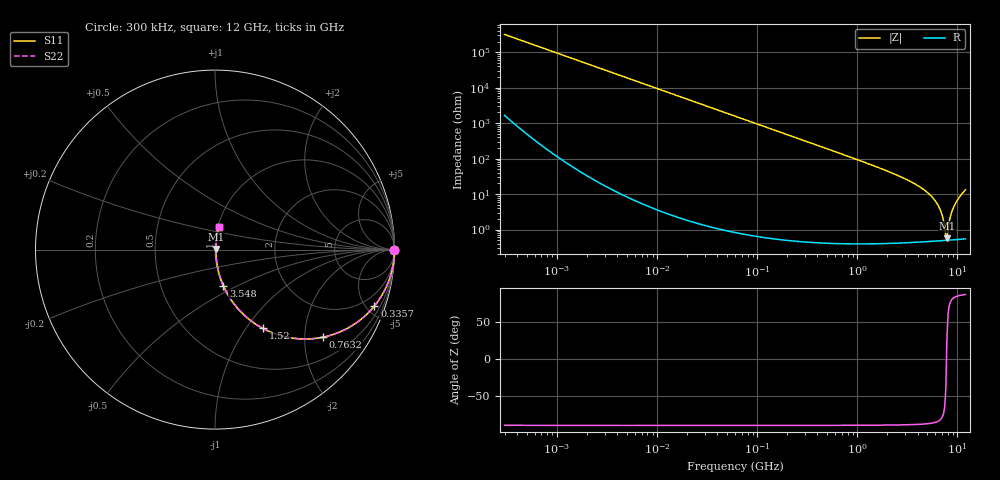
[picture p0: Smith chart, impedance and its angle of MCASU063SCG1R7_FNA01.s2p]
! MCASU063SCG1R7_FNA01  S-PARAMETER MODEL  ( General Type )
! Model Generated by TAIYO YUDEN Corporation (http://www.ty-top.com)
! Version 1.0
! TAIYO YUDEN Control No. 130801
! Copyright(c) 2013 TAIYO YUDEN CO.,LTD. All Rights Reserved.
! Product Description (link to TY-COMPAS)
! https://ds.yuden.co.jp/TYCOMPAS/or/detail?pn=MCASU063SCG1R7CFNA01&u=M
! Products Name : Multilayer Ceramic Capacitors
! Characteristics :
!  Capacitance : 1.7 pF , Rated Voltage : 50V , TCC : CG / C0G
!  Case Size : 0.6 x 0.3 / 0.024 x 0.012 [mm/inch] , Thickness : 0.3 / 0.012 [mm/inch]
!  (Conditions: Temperature = 25 degC , DC Bias Current/Voltage = 0A / 0V)
! External Node Assignments :
!  1  o---| |---o  2
! GND o---------o GND
! Frequency Range : 0.3MHz  -  12000MHz  [ 401 STEP ]
# MHz S RI R 50
! Freq[MHz].  S11 Real  S11 Imag  S21 Real  S21 Imag  S12 Real  S12 Imag  S22 Real  S22 Imag
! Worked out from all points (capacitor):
!   401 points, 300 kHz to 12 GHz, reference 50 ohm
!   read as one part in series: C = 1.68 pF near 316.3 kHz
!   lowest |Z| = 573 mohm at 7.854 GHz (marker M1)
!   series resonance near 7.772 GHz, so ESL is about 250 pH
!   S11 on the Smith chart (normalised r, x): 300 kHz: open; 335.7 MHz: 1.01, -5.64; 763.2 MHz: 1.01, -2.46; 1.52 GHz: 1.01, -1.20; 3.548 GHz: 1.01, -0.42; 12 GHz: 1.01, +0.26
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0.3  1 -0.000316  1.75e-06 0.000316  1.75e-06 0.000316  1 -0.000316
1.769972  1 -0.00187  4.88e-06 0.00187  4.88e-06 0.00187  1 -0.00187
10.44266  0.9999 -0.011  0.000125 0.011  0.000125 0.011  0.9999 -0.011
60  0.996 -0.063  0.00402 0.063  0.00402 0.063  0.996 -0.063
147.6816  0.9762 -0.152  0.0238 0.152  0.0238 0.152  0.9762 -0.152
335.7268  0.8879 -0.3147  0.1121 0.3147  0.1121 0.3147  0.8879 -0.3147
353.9943  0.8769 -0.3278  0.1231 0.3278  0.1231 0.3278  0.8769 -0.3278
763.2128  0.6021 -0.4879  0.3979 0.4879  0.3979 0.4879  0.6021 -0.4879
1519.776  0.2663 -0.4387  0.7337 0.4387  0.7337 0.4387  0.2663 -0.4387
2088.533  0.1532 -0.3554  0.8468 0.3554  0.8468 0.3554  0.1532 -0.3554
3547.679  0.0467 -0.2011  0.9533 0.2011  0.9533 0.2011  0.0467 -0.2011
4875.354  0.0181 -0.1156  0.9819 0.1156  0.9819 0.1156  0.0181 -0.1156
6026.253  0.0086 -0.0622  0.9914 0.0622  0.9914 0.0622  0.0086 -0.0622
6879.757  0.00571 -0.0298  0.9943 0.0298  0.9943 0.0298  0.00571 -0.0298
7448.838  0.00501 -0.0106  0.995 0.0106  0.995 0.0106  0.00501 -0.0106
7648.807  0.00494 -0.00422  0.9951 0.00422  0.9951 0.00422  0.00494 -0.00422
7854.144  0.00495 0.00281  0.995 -0.00281  0.995 -0.00281  0.00495 0.00281
8064.993  0.00506 0.00938  0.9949 -0.00938  0.9949 -0.00938  0.00506 0.00938
8732.115  0.00593 0.0294  0.9941 -0.0294  0.9941 -0.0294  0.00593 0.0294
9207.246  0.00703 0.0436  0.993 -0.0436  0.993 -0.0436  0.00703 0.0436
10511.28  0.0121 0.082  0.9879 -0.082  0.9879 -0.082  0.0121 0.082
12000  0.0223 0.1285  0.9777 -0.1285  0.9777 -0.1285  0.0223 0.1285
